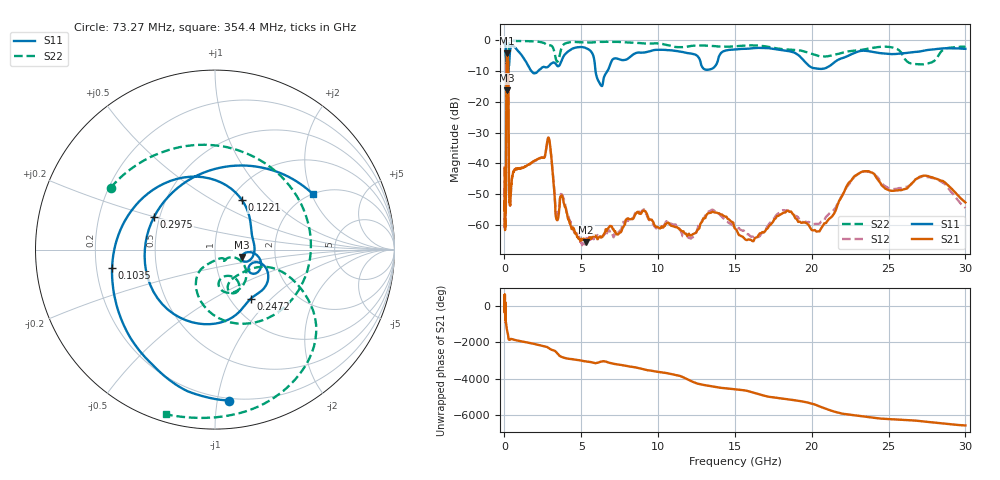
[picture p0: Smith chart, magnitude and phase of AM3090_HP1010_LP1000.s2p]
! Date/Time: Thu, Feb 28, 2019 2:04 PM
! Network Analyzer: Agilent Technologies E8364B Rev: A.07.50.67
! Sweep from 0.010 to 30.000 GHz, 1601 Points, Sweep Type: LOG
! Power Supply: 5.023 V, 0.002 A
# Hz S DB R 50
!freq MagS11 AngS11 MagS21 AngS21 MagS12 AngS12 MagS22 AngS22
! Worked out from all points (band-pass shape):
!   1601 points, 10 MHz to 30 GHz, reference 50 ohm
!   highest |S21| = -4.35 dB at 169 MHz (marker M1); lowest = -65.5 dB at 5.311 GHz (marker M2)
!   |S21| within 3 dB of the highest: 127.6 MHz to 243.2 MHz (115.6 MHz wide, 62.4 % of centre)
!   lowest |S11| = -16.3 dB at 156 MHz (marker M3), VSWR 1.36, Z = 67.1 - j5.58 ohm
!   |S11| at or under -10 dB: 122 MHz to 223.5 MHz (101.5 MHz wide, 58.8 % of centre); 1.745 GHz to 2.195 GHz (450.5 MHz wide, 22.9 % of centre); 5.927 GHz to 6.708 GHz (781.5 MHz wide, 12.4 % of centre)
!   |S22| runs from -25.1 to -0.1 dB; largest |S21 - S12| = 0.012
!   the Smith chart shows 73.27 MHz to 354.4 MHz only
!   S11 on the Smith chart (normalised r, x): 73.27 MHz: 0.18, -1.08; 103.5 MHz: 0.27, -0.08; 122.1 MHz: 1.12, +0.69; 247.2 MHz: 1.23, -0.76; 297.5 MHz: 0.47, +0.20; 354.4 MHz: 2.02, +2.05
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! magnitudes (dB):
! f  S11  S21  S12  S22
! 10 MHz  -0.3  -41.4  -41.8  -0.6
! 38.04 MHz  -0.5  -59.4  -58.9  -1.4
! 73.27 MHz  -1.5  -52.9  -55.4  -3.4
! 91.32 MHz  -3.0  -53.2  -54.3  -5.0
! 103.5 MHz  -4.7  -36.1  -35.6  -5.4
! 122.1 MHz  -10.0  -10.5  -10.5  -14.3
! 144.7 MHz  -14.0  -4.9  -4.8  -21.6
! 156 MHz  -16.3  -4.5  -4.4  -19.7
! 169 MHz  -13.4  -4.3  -4.3  -13.7
! 247.2 MHz  -9.4  -8.1  -8.1  -14.5
! 297.5 MHz  -8.3  -48.4  -49.6  -1.1
! 354.4 MHz  -4.0  -53.5  -53.8  -0.4
! 550.5 MHz  -2.0  -43.2  -43.3  -0.2
! 2.084 GHz  -10.6  -38.8  -38.9  -0.5
! 2.884 GHz  -8.4  -31.7  -31.7  -1.8
! 3.402 GHz  -8.1  -58.2  -56.5  -6.9
! 5.311 GHz  -2.6  -65.5  -65.0  -0.8
! 6.234 GHz  -14.3  -63.6  -63.9  -0.6
! 7.926 GHz  -6.3  -58.2  -58.6  -0.8
! 16.05 GHz  -2.7  -64.8  -63.8  -1.7
! 23.48 GHz  -3.5  -42.5  -42.6  -3.0
! 30 GHz  -2.8  -52.6  -54.4  -2.2
